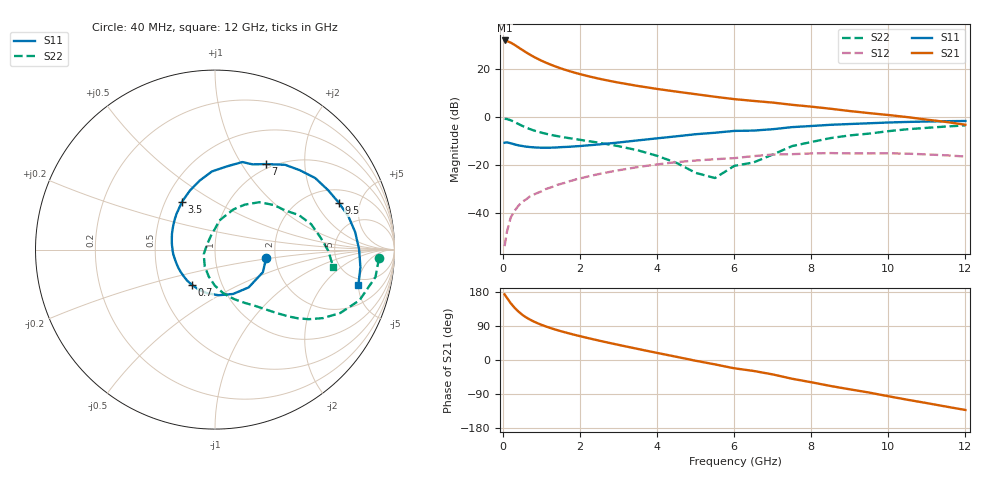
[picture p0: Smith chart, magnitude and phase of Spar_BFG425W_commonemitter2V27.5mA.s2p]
! Filename: 227bfg425.001
! BFG425W Field C1
! V1=8.688E-001V,V2=2.000E+000V, I1=3.977E-004A, I2=2.753E-002A
# GHz  S  MA  R 50
!  S11  S21  S12  S22
!Freq(GHz)  Mag  Ang  Mag  Ang  Mag  Ang  Mag  Ang
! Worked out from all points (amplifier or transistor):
!   44 points, 40 MHz to 12 GHz, reference 50 ohm
!   highest |S21| = 32.0 dB at 40 MHz (marker M1)
!   |S21| within 3 dB of that: start of sweep to 408.4 MHz
!   unconditionally stable (mu >= 1): start of sweep to 42.64 MHz; 1.094 GHz to end of sweep
!   at 700 MHz: K = 0.84, MSG = 29.6 dB, |S12| = -33.2 dB
!   at 2.4 GHz: K = 1.17, MAG = 17.7 dB, |S12| = -24.2 dB
!   at 12 GHz: K = 1.35, MAG = 3.1 dB, |S12| = -16.5 dB
!   S11 on the Smith chart (normalised r, x): 40 MHz: 1.79, -0.18; 700 MHz: 0.72, -0.30; 3.5 GHz: 0.61, +0.36; 7 GHz: 0.94, +1.29; 9.5 GHz: 2.79, +3.18; 12 GHz: 4.03, -4.96
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0.04  0.289 -9.0  39.61 173.2  0.002 72.1  0.915 -3.1
0.1  0.295 -25.3  38.56 164.1  0.004 82.3  0.907 -9.7
0.2  0.282 -48.3  35.63 149.7  0.008 76.0  0.853 -19.4
0.3  0.267 -67.8  31.96 137.8  0.011 72.1  0.782 -26.9
0.4  0.255 -85.3  28.33 127.8  0.014 68.6  0.712 -32.4
0.5  0.247 -100.6  25.09 119.2  0.017 66.4  0.651 -36.6
0.6  0.24 -112.7  22.29 112.4  0.019 65.3  0.6 -39.6
0.7  0.235 -123.0  19.96 106.6  0.022 64.1  0.557 -42.0
0.9  0.229 -140.1  16.35 96.8  0.026 62.9  0.494 -45.7
1.2  0.228 -159.0  12.72 85.4  0.033 60.9  0.43 -50.3
1.7  0.238 177.8  9.173 70.6  0.045 56.8  0.363 -57.3
2.2  0.255 160.2  7.134 58.0  0.057 51.3  0.314 -65.2
2.8  0.282 142.4  5.595 44.2  0.072 43.9  0.262 -75.7
3.5  0.324 124.5  4.441 29.1  0.09 34.0  0.201 -90.2
4.5  0.394 102.5  3.382 8.5  0.114 18.7  0.11 -121.3
5.5  0.468 82.0  2.64 -11.6  0.131 2.8  0.053 146.1
6.5  0.519 66.2  2.163 -28.9  0.152 -9.9  0.112 91.1
7  0.555 59.2  1.996 -38.1  0.164 -17.8  0.164 81.5
8.5  0.686 35.5  1.485 -68.6  0.176 -46.8  0.362 46.9
9.5  0.738 20.6  1.204 -85.9  0.173 -63.3  0.449 28.9
10.5  0.787 7.1  0.991 -105.0  0.171 -81.6  0.554 14.8
12  0.823 -14.0  0.687 -131.9  0.149 -110.8  0.667 -8.6
